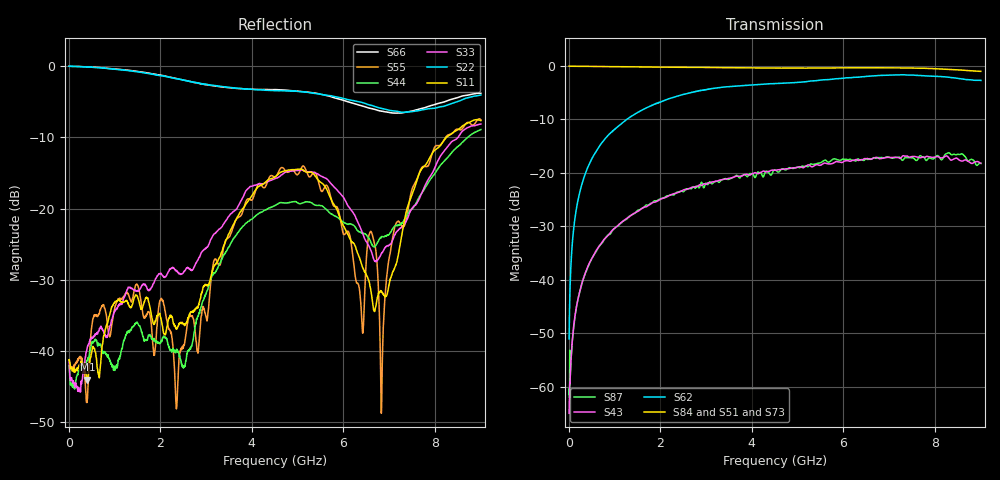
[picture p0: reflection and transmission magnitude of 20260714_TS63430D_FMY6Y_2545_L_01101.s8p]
# GHz S DB R 50
! CMT, SN0916, 25263762, 26.7.0
! Date: 15.07.2026 14:58:52
! Data: Format
! Freq S1.1:dB/Ang S1.2:dB/Ang S1.3:dB/Ang S1.4:dB/Ang S1.5:dB/Ang S1.6:dB/Ang S1.7:dB/Ang S1.8:dB/Ang
!  S2.1:dB/Ang S2.2:dB/Ang S2.3:dB/Ang S2.4:dB/Ang S2.5:dB/Ang S2.6:dB/Ang S2.7:dB/Ang S2.8:dB/Ang
!  S3.1:dB/Ang S3.2:dB/Ang S3.3:dB/Ang S3.4:dB/Ang S3.5:dB/Ang S3.6:dB/Ang S3.7:dB/Ang S3.8:dB/Ang
!  S4.1:dB/Ang S4.2:dB/Ang S4.3:dB/Ang S4.4:dB/Ang S4.5:dB/Ang S4.6:dB/Ang S4.7:dB/Ang S4.8:dB/Ang
!  S5.1:dB/Ang S5.2:dB/Ang S5.3:dB/Ang S5.4:dB/Ang S5.5:dB/Ang S5.6:dB/Ang S5.7:dB/Ang S5.8:dB/Ang
!  S6.1:dB/Ang S6.2:dB/Ang S6.3:dB/Ang S6.4:dB/Ang S6.5:dB/Ang S6.6:dB/Ang S6.7:dB/Ang S6.8:dB/Ang
!  S7.1:dB/Ang S7.2:dB/Ang S7.3:dB/Ang S7.4:dB/Ang S7.5:dB/Ang S7.6:dB/Ang S7.7:dB/Ang S7.8:dB/Ang
!  S8.1:dB/Ang S8.2:dB/Ang S8.3:dB/Ang S8.4:dB/Ang S8.5:dB/Ang S8.6:dB/Ang S8.7:dB/Ang S8.8:dB/Ang
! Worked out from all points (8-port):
!   2001 points, 10 MHz to 9 GHz, reference 50 ohm
!   strongest paths, dB at 10 MHz, 2.257 GHz, 4.505 GHz, 6.753 GHz, 9 GHz:
!     S84: -0.1, -0.3, -0.4, -0.4, -1.0
!     S51: -0.1, -0.2, -0.5, -0.4, -1.3
!     S73: -0.1, -0.3, -0.6, -0.5, -1.2
!     S62: -51.1, -6.0, -3.3, -1.8, -2.7
!     S43: -65.0, -24.0, -19.5, -17.2, -18.2
!     S87: -61.5, -24.1, -19.5, -17.2, -18.3
!   lowest |S11| = -44.0 dB at 410.1 MHz (marker M1), VSWR 1.01, Z = 50.3 - j0.573 ohm
!   |S11| at or under -10 dB: start of sweep to 8.25 GHz
